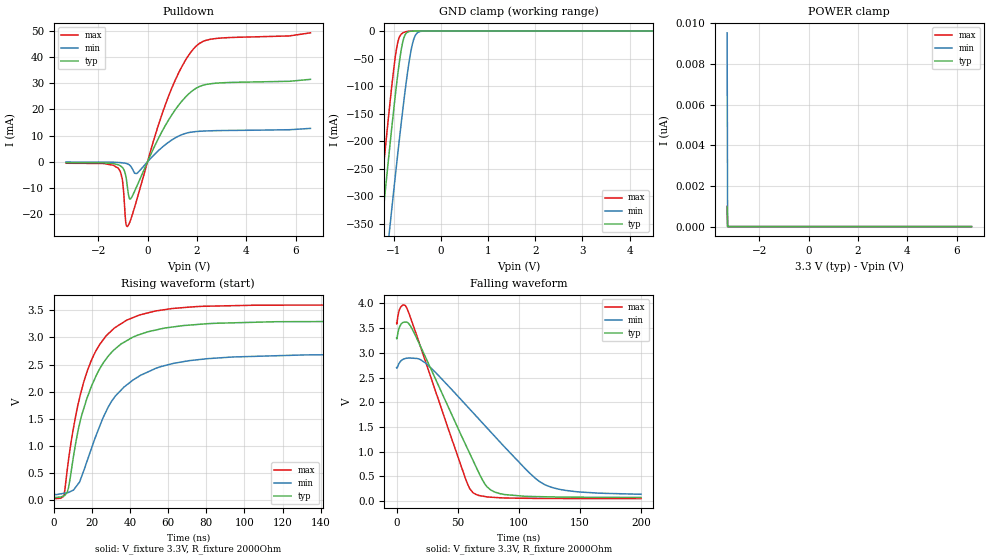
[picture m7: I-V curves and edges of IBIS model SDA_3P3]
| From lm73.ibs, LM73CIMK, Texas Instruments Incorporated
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|   (nom PVT)   (slow PVT)   (fast PVT)
|   Model SDA_3P3
[Model]   SDA_3P3
Model_type   I/O_open_drain
Polarity   Non-Inverting
Enable   Active-Low
Vinl = 0.99
Vinh = 2.31
Vmeas = 1.65
Vref = 3.3
Cref = 1pF
Rref = 2000
|   typ   min   max
|   (nom PVT)   (fast PVT)   (slow PVT)
C_comp   0.724p   0.674p   0.794p
|C_comp (ON state)   0.809p   0.769p   0.824p
|C_comp (OFF state)   0.724p   0.674p   0.794p
[Model spec]
|subparameter
Vinl   0.99   0.81   1.08
Vinh   2.31   1.89   2.52
[Voltage Range]   3.3   2.7   3.6
[Temperature Range]   27   150   -40
[Pullup Reference]   3.3   2.7   3.6
[Pulldown Reference]   0   0   0
[Power Clamp Reference]   3.3   2.7   3.6
[GND Clamp Reference]   0   0   0
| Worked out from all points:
|   slope of the pulldown table from 0 to 0.495 V, typ, clamps not added: 50 ohm
|   GND clamp passes 1 mA (typ) near -0.68 V on its own axis
|   falling waveform, V_fixture 3.3V, R_fixture 2000Ohm: 20-80 % time 36.1ns typ, 57.7ns min, 29.4ns max; typ from 3.3 V to 0.075 V
|   rising waveform, V_fixture 3.3V, R_fixture 2000Ohm: 20-80 % time 18.6ns typ, 23.7ns min, 16.7ns max; typ from 0.074 V to 3.3 V
[Pulldown]
|   Voltage   I(typ)   I(min)   I(max)
-3.3V     -353.1uA   -104.8uA   -552uA
-1.191V   -1.131mA   -257.5uA   -2.421mA
-1.023V   -2.11mA    -378uA     -6.565mA
-884.4mV  -5.177mA   -584.5uA   -22.86mA
-815.1mV  -9.548mA   -777.4uA   -24.76mA
-676.5mV  -14.09mA   -1.718mA   -22.01mA
-429mV    -9.265mA   -4.432mA   -14.32mA
848.1mV   15.89mA    7.459mA    24.97mA
1.403V    23.3mA     10.41mA    36.57mA
1.957V    28.05mA    11.55mA    44.1mA
2.788V    30.05mA    11.9mA     47.14mA
6.6V      31.52mA    12.76mA    49.29mA
[GND Clamp]
|   Voltage   I(typ)   I(min)   I(max)
-3.3V     -2.187A    -2.243A    -2.165A
-1.379V   -462.3mA   -601.4mA   -389.9mA
-1.29V    -384.4mA   -526.6mA   -310.1mA
-1.201V   -307.5mA   -452.4mA   -231.7mA
-1.112V   -232.1mA   -379.1mA   -155.7mA
-1.053V   -183.2mA   -330.8mA   -107.5mA
-924mV    -84.35mA   -228.8mA   -23.8mA
-844.8mV  -35.15mA   -168.7mA   -5.889mA
-785.4mV  -12.1mA    -125.8mA   -2.451mA
-607.2mV  -151.7uA   -24.38mA   -45.94uA
-438.9mV  -1.197uA   -749.5uA   -115.4nA
6.6V      0A         0A         0A
[POWER Clamp]
|   Voltage   I(typ)   I(min)   I(max)
-3.3V     965.2pA    9.534nA    1.007nA
-3.28V    0A         0A         0A
-3.27V    0A         0A         0A
6.6V      0A         0A         0A
[Ramp]
R_load = 2000
|   typ   min   max
dV/dt_r   1.93565/1.85843e-08   1.54305/2.36184e-08   2.12962/1.66459e-08
dV/dt_f   1.93486/3.60119e-08   1.53581/5.77478e-08   2.12936/2.92613e-08
[Falling Waveform]
V_fixture = 3.3V
V_fixture_min = 2.7V
V_fixture_max = 3.6V
R_fixture = 2000Ohm
C_fixture = 0F
|   Time   V(typ)   V(min)   V(max)
0s        3.3V       2.7V       3.6V
3.471ns   3.571V     2.836V     3.931V
8.927ns   3.612V     2.892V     3.873V
23.78ns   2.906V     2.792V     2.815V
56.78ns   1.126V     1.944V     429.2mV
63.23ns   787.3mV    1.771V     161.2mV
72.41ns   341.8mV    1.524V     93.9mV
80.38ns   184.1mV    1.309V     76.44mV
121.8ns   89.83mV    328.5mV    55.07mV
199.9ns   75.24mV    140.3mV    51.07mV
[Rising Waveform]
V_fixture = 3.3V
V_fixture_min = 2.7V
V_fixture_max = 3.6V
R_fixture = 2000Ohm
C_fixture = 0F
|   Time   V(typ)   V(min)   V(max)
0s        73.64mV    123.9mV    50.62mV
5.23ns    78.1mV     125.1mV    85.96mV
7.057ns   147mV      136.3mV    563.1mV
12.54ns   1.249V     288.2mV    1.738V
19.53ns   2.08V      931.3mV    2.564V
28.58ns   2.657V     1.72V      3.068V
38.15ns   2.939V     2.122V     3.317V
54.84ns   3.148V     2.447V     3.496V
80.66ns   3.254V     2.609V     3.576V
199.9ns   3.3V       2.696V     3.6V
